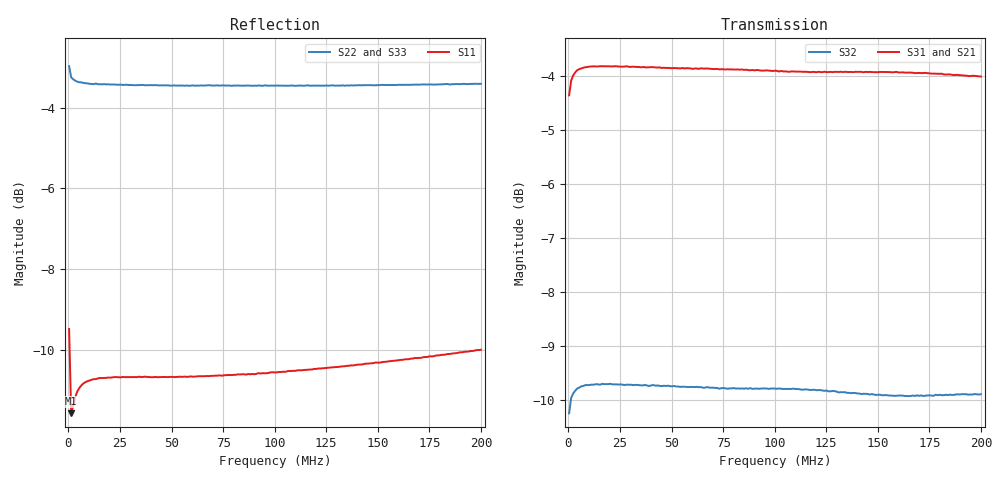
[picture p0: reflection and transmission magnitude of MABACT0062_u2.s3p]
#	MHz	S	RI	R	50
!FREQ	R1	I1	R2	I2	R3	I3
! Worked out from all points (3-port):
!   201 points, 300 kHz to 200 MHz, reference 50 ohm
!   strongest paths, dB at 300 kHz, 50.23 MHz, 100.2 MHz, 150.1 MHz, 200 MHz:
!     S31: -4.4, -3.9, -3.9, -3.9, -4.0
!     S21: -4.5, -3.9, -3.9, -4.1, -4.1
!     S32: -10.2, -9.7, -9.8, -9.9, -9.9
!   lowest |S11| = -11.6 dB at 1.298 MHz (marker M1), VSWR 1.72, Z = 80.9 + j16 ohm
!   |S11| at or under -10 dB: 546.2 kHz to 199.9 MHz (199.4 MHz wide, 199 % of centre)
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0.3  0.1621 0.2938  0.5858 0.1478  -0.5869 -0.1473
     0.5804 0.1461  -0.7061 0.0748  -0.299 -0.0759
     -0.5869 -0.1473  -0.2981 -0.0756  -0.7057 0.0739
1.2985  0.2473 0.0919  0.623 0.0446  -0.623 -0.0442
        0.6232 0.0453  -0.6872 0.025  -0.3174 -0.0226
        -0.623 -0.0442  -0.317 -0.0226  -0.687 0.0253
2.297  0.2614 0.0659  0.6304 0.0306  -0.6306 -0.0307
       0.6304 0.0311  -0.6835 0.0204  -0.3213 -0.0157
       -0.6306 -0.0307  -0.3205 -0.0155  -0.6833 0.0208
5.2925  0.2809 0.0393  0.6395 0.0168  -0.6396 -0.0166
        0.6396 0.0165  -0.6779 0.0182  -0.3262 -0.00896
        -0.6396 -0.0166  -0.3247 -0.00873  -0.6776 0.019
9.2865  0.288 0.0265  0.6429 0.00839  -0.6428 -0.00815
        0.6425 0.00864  -0.6756 0.0209  -0.3275 -0.00478
        -0.6428 -0.00815  -0.3265 -0.00502  -0.6752 0.0217
17.2745  0.2912 0.0189  0.6444 0.00165  -0.6439 -0.00125
         0.6438 0.00177  -0.6739 0.0301  -0.3282 -0.0016
         -0.6439 -0.00125  -0.3273 -0.00145  -0.6734 0.0312
42.237  0.2921 0.0185  0.642 -0.00739  -0.6422 0.00934
        0.6419 -0.00919  -0.6697 0.0632  -0.3272 0.0025
        -0.6422 0.00934  -0.3261 0.00316  -0.6681 0.0677
100.15  0.2943 0.0354  0.6358 -0.0194  -0.6372 0.0244
        0.6358 -0.0206  -0.6562 0.1429  -0.3252 0.00739
        -0.6372 0.0244  -0.324 0.00728  -0.6511 0.1501
160.06  0.3021 0.0541  0.6292 -0.0294  -0.6343 0.036
        0.6233 -0.0301  -0.6357 0.2219  -0.3206 0.0098
        -0.6343 0.036  -0.3192 0.0104  -0.6244 0.2314
200  0.3094 0.0657  0.6201 -0.0355  -0.6283 0.0435
     0.6228 -0.0377  -0.618 0.2721  -0.3214 0.0137
     -0.6283 0.0435  -0.32 0.013  -0.602 0.2817
